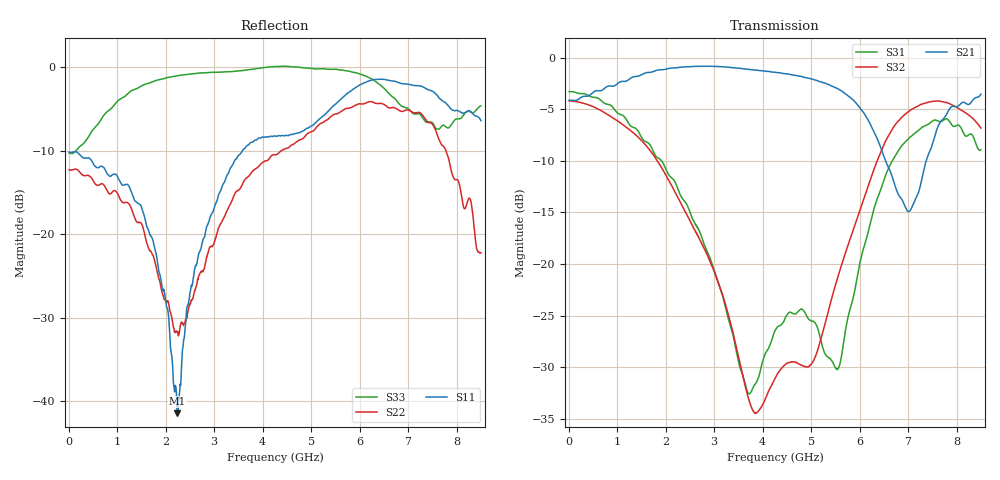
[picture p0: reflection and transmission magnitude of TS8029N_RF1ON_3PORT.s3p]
!Created with skrf (http://scikit-rf.org).
# GHz S RI R 50.0
!freq ReS11 ImS11 ReS12 ImS12 ReS13 ImS13
! ReS21 ImS21 ReS22 ImS22 ReS23 ImS23
! ReS31 ImS31 ReS32 ImS32 ReS33 ImS33
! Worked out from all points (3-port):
!   1601 points, 10 MHz to 8.5 GHz, reference 50 ohm
!   strongest paths, dB at 10 MHz, 2.132 GHz, 4.255 GHz, 6.378 GHz, 8.5 GHz:
!     S21: -4.1, -1.0, -1.4, -8.0, -3.5
!     S32: -4.2, -12.5, -31.1, -9.8, -6.8
!     S31: -3.3, -11.7, -26.5, -13.5, -8.9
!   lowest |S11| = -41.4 dB at 2.244 GHz (marker M1), VSWR 1.02, Z = 49.2 + j0.0828 ohm
!   |S11| at or under -10 dB: start of sweep to 3.582 GHz
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0.01  -0.3105 0.00409  0.623 0.000261  0.6861 -0.00735
      0.623 0.000213  -0.2433 0.00307  0.6187 -0.00785
      0.686 -0.00749  0.6187 -0.00777  -0.3065 0.0118
0.9704312  -0.1566 0.1664  0.7312 -0.0964  0.3004 -0.462
           0.7317 -0.0965  -0.082 0.1617  0.2424 -0.4382
           0.3003 -0.4626  0.2426 -0.4378  0.383 0.4737
2.243931  -0.00843 0.000842  0.7049 -0.552  -0.1083 -0.2081
          0.7047 -0.5523  0.0186 -0.0184  -0.1516 -0.1484
          -0.1081 -0.2083  -0.1513 -0.1488  0.7463 -0.4808
2.8966  -0.0704 -0.0973  0.5156 -0.7491  -0.0816 -0.0733
        0.5157 -0.7497  -0.0747 -0.0338  -0.1025 -0.0257
        -0.0816 -0.0735  -0.1024 -0.0256  0.3663 -0.8532
3.708456  -0.2836 -0.1919  0.1867 -0.8601  -0.00477 -0.0231
          0.1859 -0.8601  -0.2208 -0.0266  -0.00757 0.0211
          -0.00479 -0.023  -0.00753 0.021  -0.3897 -0.8828
4.255  -0.348 -0.1695  -0.0398 -0.8496  0.0258 -0.0399
       -0.0406 -0.8489  -0.2954 0.0434  0.0265 0.0087
       0.0256 -0.04  0.0265 0.00873  -0.6167 -0.7959
5.555031  -0.6026 0.1436  -0.45 -0.5455  -0.03 0.00767
          -0.4508 -0.545  -0.1695 0.5012  0.0654 0.058
          -0.03 0.00774  0.0653 0.0581  -0.9169 0.3043
6.446481  -0.5505 0.6428  -0.33 -0.1462  0.1486 0.1803
          -0.3308 -0.1464  0.193 0.5752  0.3493 0.0583
          0.1486 0.1806  0.3485 0.0584  -0.4056 0.6594
7.544875  0.1422 0.6876  -0.0271 -0.4107  0.3196 -0.3819
          -0.0273 -0.4109  0.4262 -0.0795  0.08 -0.6105
          0.3197 -0.3833  0.0809 -0.6103  0.269 0.352
8.5  0.1783 0.444  -0.3862 -0.544  -0.1869 -0.3056
     -0.3874 -0.5429  0.046 -0.0622  -0.3973 -0.2234
     -0.1875 -0.3055  -0.3974 -0.2247  0.5856 0.00664
